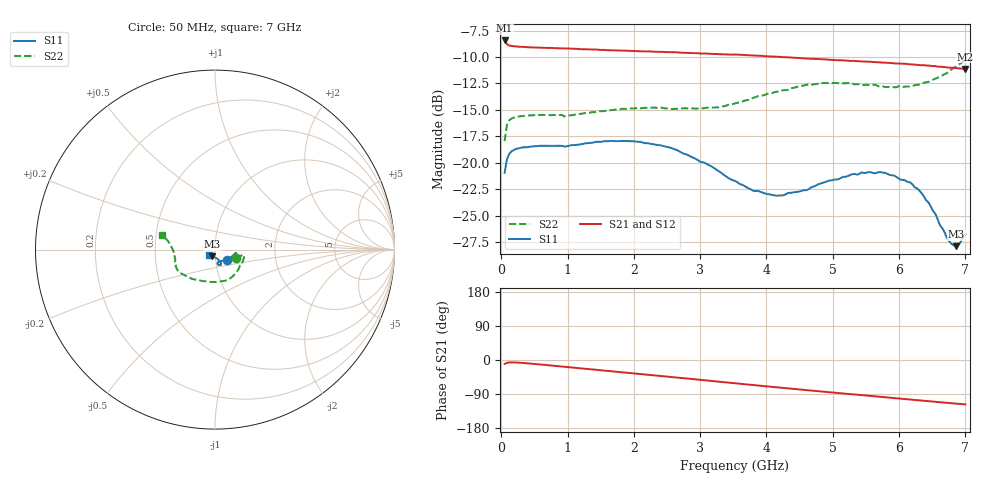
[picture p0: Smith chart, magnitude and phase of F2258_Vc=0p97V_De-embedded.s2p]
! Integrated Device Technology
! Corporate Headquarters
! 6024 Silver Creek Valley Road
! San Jose, CA 95138  USA
! Phone:  1-408-284-8200
! Toll Free:  1-800-223-1366
! Webpage:  http://www.idt.com/
! Timing and RF Division
! 515 Groton Road, Suite 102
! Westford, MA 01886-6024
! Device:  F2258
! Description: Voltage Variable RF Attenuator
! Frequency:  50.0 -  6000.00 MHz
! Package:  3x3 mm Thin QFN Plastic Package: 16 pin
! Ports:  2 RF, 2 DC
!  Pin  1  = NC
!  Pin  2  = NC
!  Pin  3  = RF2  = Port 2
!  Pin  4  = GND
!  Pin  5  = Vdd
!  Pin  6  = NC
!  Pin  7  = VCTRL
!  Pin  8  = NC
!  Pin  9  = GND
!  Pin 10  = RF1  = Port 1
!  Pin 11  = NC
!  Pin 12  = NC
!  Pin 13  = NC
!  Pin 14  = NC
!  Pin 15  = NC
!  Pin 16  = NC
! Vcntrl:  0.970 Volts
! Vdd:  +3.300 Volts
! Current:  1.152 mA
! Data:  The device was measured on a the F2258 evaluation board which has
!  individual transmission lines to the RF pins.  Data was collected
!  using a calibrated network analyzer.  The evaluation board was
!  de-embedded using a TRL calibration technique.
!  The reference plane is the edge of the package pin.
! Misc:  SN 10
!  Action Tracker AT0285
! Date Measured:  2014-12-10
! Date:  2016-01-13  MJV
! Note:
!  Integrated Device Technology supplies this data as a sample of measured
!  data at the package pin for this product.  Your particular data for this
!  product may vary.
!  Data was taken at 25 degrees C.
!  Integrated Device Technology reserves the right to change this data at anytime.
!Freq_(GHz)  S11M_(dB)  S11P_(deg)  S21M_(dB)  S21P_(deg)  S12M_(dB)  S12P_(deg)  S22M_(dB)  S22P_(deg)
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# GHz S dB R 50
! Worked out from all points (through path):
!   201 points, 50 MHz to 7 GHz, reference 50 ohm
!   highest |S21| = -8.44 dB at 50 MHz (marker M1); lowest = -11.1 dB at 7 GHz (marker M2)
!   group delay of S21, straight-line fit = 45.9 ps
!   lowest |S11| = -27.9 dB at 6.861 GHz (marker M3), VSWR 1.08, Z = 48.3 - j3.6 ohm
!   |S11| at or under -10 dB: start of sweep to end of sweep
!   |S22| runs from -17.9 to -10.2 dB; largest |S21 - S12| = 0.0015
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0.05  -20.95 -41.4  -8.44 -10.3  -8.43 -10.3  -17.94 -22.9
0.08475  -19.67 -20.2  -8.79 -7.4  -8.80 -7.4  -16.43 -12.6
0.1195  -19.15 -13.7  -8.92 -6.5  -8.93 -6.5  -15.98 -10.6
0.189  -18.78 -9.8  -8.99 -6.4  -9.00 -6.4  -15.72 -10.4
1.2315  -18.21 -19.9  -9.27 -22.6  -9.28 -22.6  -15.33 -41.4
1.89175  -17.93 -24.1  -9.41 -33.6  -9.44 -33.6  -14.91 -59.2
2.37825  -18.32 -26.8  -9.51 -41.7  -9.50 -41.7  -14.79 -72.8
2.65625  -18.81 -29.4  -9.56 -46.4  -9.55 -46.4  -14.89 -81.4
3.07325  -20.01 -34.9  -9.67 -53.6  -9.65 -53.6  -14.83 -96.6
3.525  -21.70 -46.5  -9.77 -61.4  -9.77 -61.4  -14.39 -114.8
3.803  -22.64 -57.7  -9.87 -66.1  -9.88 -66.1  -13.85 -125.3
4.1505  -23.10 -69.5  -9.98 -72.0  -9.98 -72.0  -13.28 -135.7
4.7065  -22.25 -79.6  -10.17 -81.2  -10.17 -81.2  -12.60 -148.3
5.43625  -20.90 -73.8  -10.42 -92.8  -10.42 -92.7  -12.64 -159.9
5.71425  -20.87 -68.5  -10.51 -97.2  -10.50 -97.1  -12.80 -165.1
5.85325  -21.13 -67.6  -10.56 -99.3  -10.57 -99.4  -12.82 -168.5
6.166  -21.84 -65.9  -10.69 -104.3  -10.70 -104.3  -12.81 -175.8
6.305  -22.61 -66.6  -10.76 -106.5  -10.77 -106.5  -12.60 -179.5
6.54825  -24.83 -73.0  -10.86 -110.4  -10.88 -110.3  -12.05 174.2
6.722  -27.09 -88.0  -10.98 -113.0  -10.99 -113.0  -11.52 169.6
6.861  -27.86 -113.2  -11.05 -115.1  -11.06 -115.1  -10.89 167.0
7  -26.74 -141.3  -11.14 -117.1  -11.15 -117.1  -10.23 164.3
